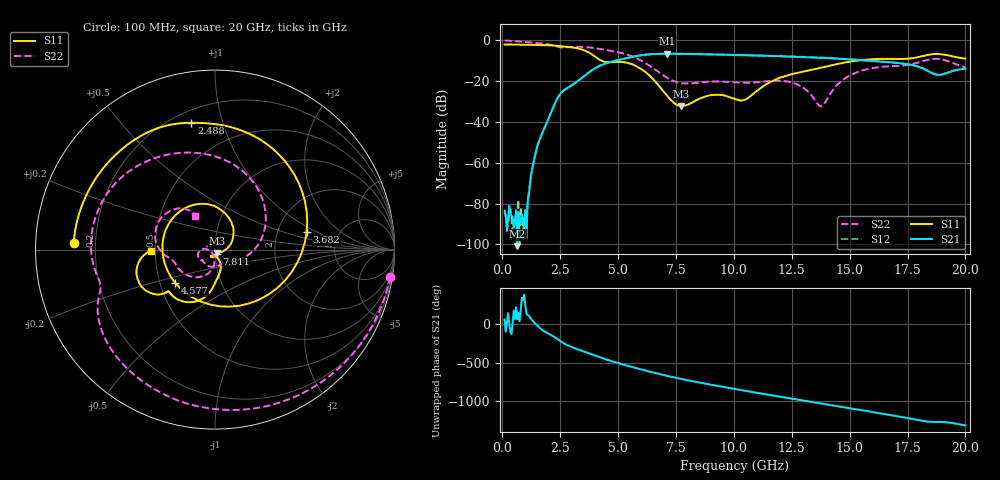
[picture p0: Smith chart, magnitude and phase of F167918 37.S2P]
!  2-Port S-parameters saved by WinCal
! VAR MeasName=S-Parameters (CALIBRATED_DATA) read from VNA (N5242A)
! VAR MeasDate=2016-11-22 10:26:32
! VAR NAME=F167918 37
! VAR FILENAME=F167918 37.S2P
! VAR DATE=2016-11-22 10:26:32
! VAR PHYS_PORTS=1,2
# Hz S DB R 50
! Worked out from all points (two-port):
!   401 points, 100 MHz to 20 GHz, reference 50 ohm
!   highest |S21| = -6.59 dB at 7.115 GHz (marker M1); lowest = -100.9 dB at 647.2 MHz (marker M2)
!   |S21| within 3 dB of the highest: 5.043 GHz to 15.27 GHz (10.22 GHz wide, 101 % of centre)
!   lowest |S11| = -32.2 dB at 7.712 GHz (marker M3), VSWR 1.05, Z = 51.2 - j2.16 ohm
!   |S11| at or under -10 dB: 4.283 GHz to 15.31 GHz (11.03 GHz wide, 113 % of centre)
!   |S22| runs from -32.5 to -0.1 dB; largest |S21 - S12| = 0.0049
!   S11 on the Smith chart (normalised r, x): 100 MHz: 0.12, +0.02; 2.488 GHz: 0.27, +0.79; 3.682 GHz: 2.93, +0.79; 4.577 GHz: 0.60, -0.24; 7.811 GHz: 1.02, -0.05; 20 GHz: 0.47, -0.01
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1e8  -2.07 177.3  -84.63 63.8  -82.99 27.5  -0.10 -8.8
6.4725e8  -2.14 162.7  -100.88 66.4  -84.90 80.7  -0.49 -52.4
1.04525e9  -2.21 151.8  -97.05 139.7  -91.25 154.5  -0.88 -81.2
1.54275e9  -2.32 137.0  -50.86 -25.1  -50.84 -25.1  -1.43 -113.0
2.488e9  -2.87 100.5  -26.52 147.6  -26.53 147.3  -3.43 -161.2
3.43325e9  -4.50 38.3  -18.46 18.4  -18.48 18.5  -3.26 161.5
3.682e9  -5.68 10.9  -16.25 -8.0  -16.26 -7.8  -3.45 149.8
4.12975e9  -8.98 -57.5  -12.96 -57.2  -12.92 -57.2  -4.09 128.6
4.5775e9  -10.78 -140.2  -10.99 -103.9  -10.93 -104.2  -4.92 107.7
5.672e9  -12.04 95.3  -7.97 161.1  -7.99 160.7  -8.19 47.7
6.7665e9  -22.32 11.0  -6.64 75.6  -6.67 75.6  -15.73 -16.6
7.11475e9  -27.12 -14.6  -6.59 51.2  -6.62 51.2  -18.37 -31.3
7.71175e9  -32.22 -59.2  -6.65 12.2  -6.66 12.2  -20.99 -51.2
7.81125e9  -32.12 -64.5  -6.67 5.9  -6.67 6.0  -21.11 -54.7
9.00525e9  -26.91 -109.8  -6.95 -63.9  -6.93 -64.0  -20.23 -101.6
1.005e10  -28.81 -116.4  -7.20 -120.8  -7.22 -120.7  -20.63 -131.3
1.149275e10  -20.93 -69.4  -7.63 164.7  -7.62 164.8  -20.08 -147.1
1.338325e10  -14.40 -90.4  -8.37 69.9  -8.31 70.2  -27.36 177.6
1.378125e10  -13.42 -93.6  -8.56 50.2  -8.50 50.3  -32.46 -137.7
1.49255e10  -10.63 -106.8  -9.34 -6.6  -9.25 -6.8  -17.74 -103.7
1.67165e10  -9.14 -133.8  -10.74 -95.9  -10.73 -96.3  -12.78 -154.3
2e10  -8.96 -179.1  -13.93 125.7  -13.91 125.0  -13.24 120.5
